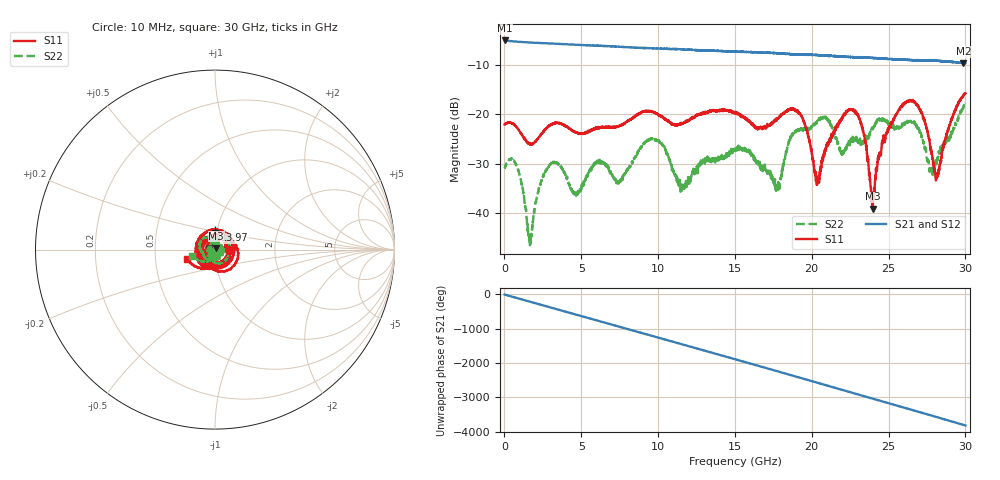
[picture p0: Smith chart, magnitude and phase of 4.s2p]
#  HZ  S  DB  R  50.00
! Rohde & Schwarz Vector Network Analyzer
! Rohde-Schwarz,ZNB40-4Port,1311601084101679,3.45
! Created: UTC 10/20/2022, 5:23:49 PM
! freq[Hz]  db:S11  ang:S11  db:S31  ang:S31  db:S13  ang:S13  db:S33  ang:S33
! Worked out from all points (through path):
!   3000 points, 10 MHz to 30 GHz, reference 50 ohm
!   highest |S21| = -4.95 dB at 20 MHz (marker M1); lowest = -9.6 dB at 29.87 GHz (marker M2)
!   group delay of S21, straight-line fit = 353 ps
!   lowest |S11| = -39.2 dB at 23.98 GHz (marker M3), VSWR 1.02, Z = 50.7 + j0.868 ohm
!   |S11| at or under -10 dB: start of sweep to end of sweep
!   |S22| runs from -46.8 to -17.7 dB; largest |S21 - S12| = 0.01
!   S11 on the Smith chart (normalised r, x): 10 MHz: 1.17, -0.00; 13.97 GHz: 0.98, +0.21; 30 GHz: 0.73, -0.08
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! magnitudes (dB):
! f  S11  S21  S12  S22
! 10 MHz  -22.0  -5.0  -5.0  -30.9
! 20 MHz  -21.9  -4.9  -5.0  -30.9
! 840 MHz  -22.8  -5.2  -5.2  -30.9
! 1.66 GHz  -26.0  -5.4  -5.4  -46.6
! 3.01 GHz  -22.1  -5.6  -5.6  -30.1
! 5.01 GHz  -23.9  -5.9  -5.9  -34.7
! 10.01 GHz  -20.0  -6.6  -6.6  -25.3
! 11.58 GHz  -21.8  -6.8  -6.8  -35.1
! 13.97 GHz  -19.4  -7.1  -7.1  -28.8
! 15.01 GHz  -19.5  -7.2  -7.2  -27.0
! 17.77 GHz  -20.8  -7.5  -7.5  -34.8
! 19.14 GHz  -19.5  -7.8  -7.8  -23.3
! 20.01 GHz  -28.2  -7.8  -7.9  -22.3
! 20.42 GHz  -33.7  -7.9  -7.9  -21.4
! 22.73 GHz  -19.1  -8.3  -8.3  -24.9
! 23.36 GHz  -23.6  -8.4  -8.4  -25.3
! 23.98 GHz  -39.2  -8.5  -8.5  -22.9
! 25.01 GHz  -23.0  -8.7  -8.6  -22.2
! 26.72 GHz  -17.5  -9.0  -8.9  -22.1
! 28.15 GHz  -32.3  -9.0  -9.0  -29.5
! 29.87 GHz  -16.2  -9.6  -9.5  -18.4
! 30 GHz  -15.7  -9.6  -9.6  -17.7
